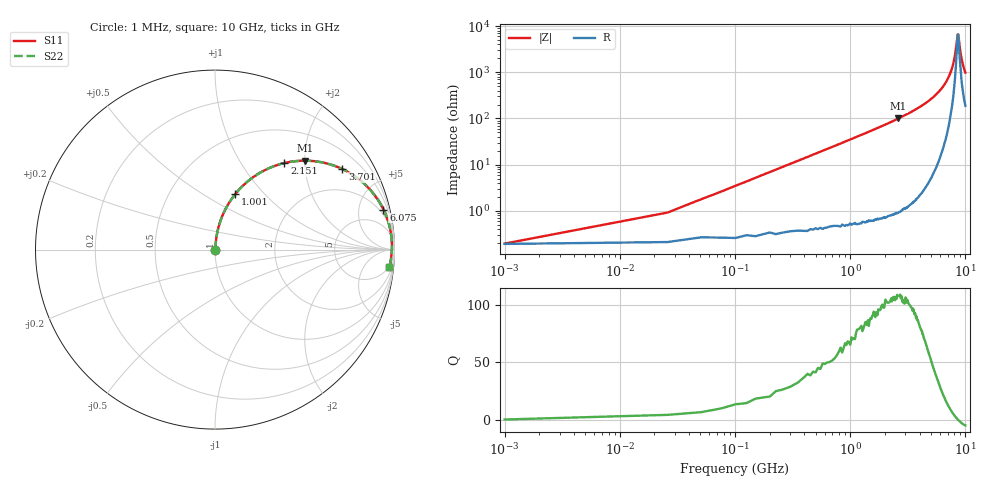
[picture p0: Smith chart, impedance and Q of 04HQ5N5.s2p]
! Coilcraft 0403HQ-5N5 Chip Inductor
! 13 February 2004
# MHZ S MA R 50
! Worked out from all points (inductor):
!   401 points, 1 MHz to 10 GHz, reference 50 ohm
!   read as one part in series: L = 5.51 nH near 50.99 MHz
!   highest Q = 108 at 2.626 GHz (marker M1), where L = 6.06 nH
!   self-resonance near 8.626 GHz
!   S11 on the Smith chart (normalised r, x): 1 MHz: 1.00, +0.00; 1.001 GHz: 1.01, +0.70; 2.151 GHz: 1.02, +1.58; 3.701 GHz: 1.03, +3.14; 6.075 GHz: 1.32, +8.32; 10 GHz: 5, -19
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1  0.001891 10.5  0.998 -0.0  0.998 -0.0  0.001891 10.5
75.992  0.026 82.7  0.997 -1.5  0.997 -1.5  0.026 82.7
100.99  0.035 83.4  0.997 -2.0  0.997 -2.0  0.035 83.4
150.985  0.052 83.7  0.996 -3.0  0.996 -3.0  0.052 83.7
225.977  0.078 83.1  0.994 -4.5  0.994 -4.5  0.078 83.1
525.947  0.179 78.4  0.98 -10.3  0.98 -10.3  0.179 78.4
1000.9  0.329 69.9  0.939 -19.2  0.939 -19.2  0.329 69.9
1675.832  0.513 58.5  0.853 -30.9  0.853 -30.9  0.513 58.5
2150.785  0.618 51.3  0.78 -38.2  0.78 -38.2  0.618 51.3
2625.737  0.704 44.7  0.704 -44.7  0.704 -44.7  0.704 44.7
3350.665  0.803 36.0  0.588 -53.4  0.588 -53.4  0.803 36.0
3700.63  0.839 32.3  0.535 -57.0  0.535 -57.0  0.839 32.3
5000.5  0.928 20.9  0.356 -68.0  0.356 -68.0  0.928 20.9
6075.393  0.964 13.4  0.231 -74.5  0.231 -74.5  0.964 13.4
6675.333  0.976 9.8  0.17 -77.0  0.17 -77.0  0.976 9.8
7775.223  0.985 3.9  0.07 -76.0  0.07 -76.0  0.985 3.9
8125.188  0.986 2.3  0.042 -69.3  0.042 -69.3  0.986 2.3
8350.165  0.986 1.2  0.025 -56.1  0.025 -56.1  0.986 1.2
8525.148  0.986 0.4  0.016 -28.1  0.016 -28.1  0.986 0.4
8650.135  0.985 -0.1  0.015 7.1  0.015 7.1  0.985 -0.1
9300.07  0.982 -2.8  0.052 68.7  0.052 68.7  0.982 -2.8
10000  0.976 -5.6  0.099 73.4  0.099 73.4  0.976 -5.6
